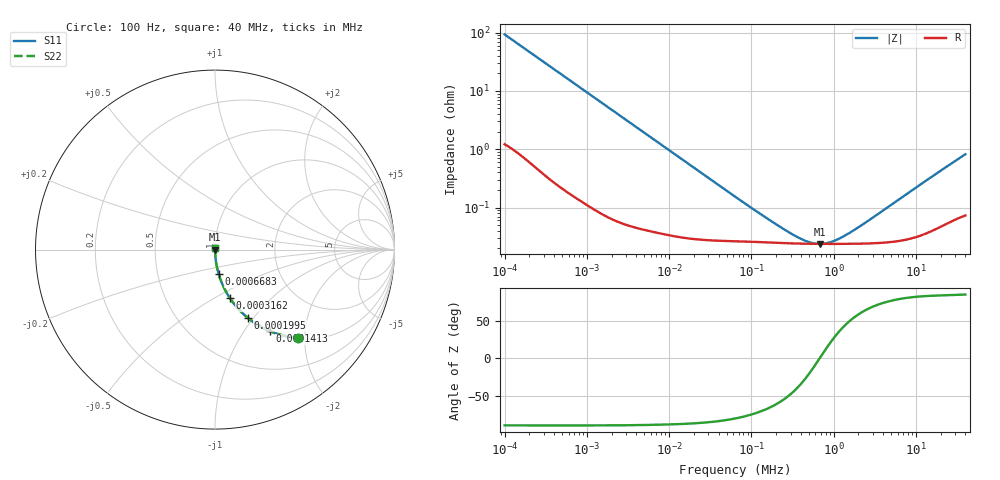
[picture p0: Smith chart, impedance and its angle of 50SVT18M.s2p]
!  *** S-Parameter ***
!  Copyright (C) Panasonic Industry
!  Conductive Polymer Aluminum Solid Capacitors (OS-CON)
!  Parts No. 50SVT18M
! Touchstone file from project
# GHZ S RI R 50.000000
! Modal data exported
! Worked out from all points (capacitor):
!   450 points, 100 Hz to 40 MHz, reference 50 ohm
!   read as one part in series: C = 17.1 uF near 105.9 Hz
!   lowest |Z| = 23.8 mohm at 687.9 kHz (marker M1)
!   series resonance near 676.2 kHz, so ESL is about 3.2 nH
!   S11 on the Smith chart (normalised r, x): 100 Hz: 1.02, -1.86; 141.3 Hz: 1.02, -1.32; 199.5 Hz: 1.01, -0.94; 316.2 Hz: 1.01, -0.59; 668.3 Hz: 1.00, -0.28; 40 MHz: 1.00, +0.02
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1e-07  0.464 -0.4922  0.536 0.4922  0.536 0.4922  0.464 -0.4922
1.412538e-07  0.3062 -0.4543  0.6938 0.4543  0.6938 0.4543  0.3062 -0.4543
1.995262e-07  0.1836 -0.3809  0.8164 0.3809  0.8164 0.3809  0.1836 -0.3809
2.511886e-07  0.1254 -0.3252  0.8746 0.3252  0.8746 0.3252  0.1254 -0.3252
3.162278e-07  0.0838 -0.2713  0.9162 0.2713  0.9162 0.2713  0.0838 -0.2713
4.466836e-07  0.0446 -0.2009  0.9554 0.2009  0.9554 0.2009  0.0446 -0.2009
6.683439e-07  0.0211 -0.138  0.9789 0.138  0.9789 0.138  0.0211 -0.138
8.659643e-07  0.013 -0.1076  0.987 0.1076  0.987 0.1076  0.013 -0.1076
2.113489e-06  0.00262 -0.0448  0.9974 0.0448  0.9974 0.0448  0.00262 -0.0448
7.498942e-06  0.000525 -0.0127  0.9995 0.0127  0.9995 0.0127  0.000525 -0.0127
6.493816e-05  0.000265 -0.00148  0.9997 0.00148  0.9997 0.00148  0.000265 -0.00148
0.0001496236  0.000253 -0.000624  0.9997 0.000624  0.9997 0.000624  0.000253 -0.000624
0.0002818383  0.000244 -0.000292  0.9998 0.000292  0.9998 0.000292  0.000244 -0.000292
0.0004097321  0.00024 -0.000155  0.9998 0.000155  0.9998 0.000155  0.00024 -0.000155
0.0005463865  0.000238 -6.38e-05  0.9998 6.38e-05  0.9998 6.38e-05  0.000238 -6.38e-05
0.0006878599  0.000238 5.13e-06  0.9998 -5.13e-06  0.9998 -5.13e-06  0.000238 5.13e-06
0.0009440609  0.000237 0.000101  0.9998 -0.000101  0.9998 -0.000101  0.000237 0.000101
0.001333521  0.000238 0.000218  0.9998 -0.000218  0.9998 -0.000218  0.000238 0.000218
0.002113489  0.00024 0.000417  0.9998 -0.000417  0.9998 -0.000417  0.00024 0.000417
0.004731513  0.000255 0.00102  0.9997 -0.00102  0.9997 -0.00102  0.000255 0.00102
0.01584893  0.00041 0.0034  0.9996 -0.0034  0.9996 -0.0034  0.00041 0.0034
0.04  0.000796 0.00816  0.9992 -0.00816  0.9992 -0.00816  0.000796 0.00816
